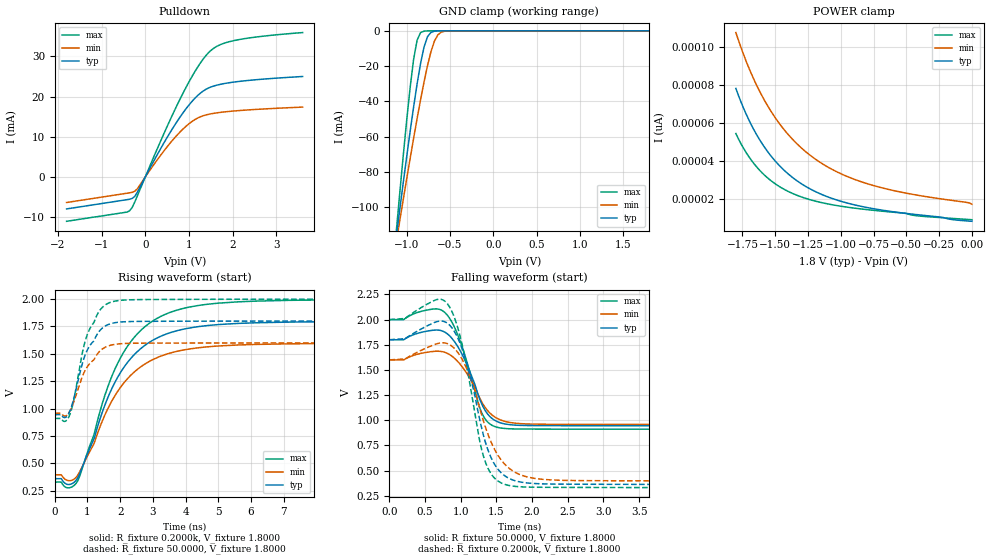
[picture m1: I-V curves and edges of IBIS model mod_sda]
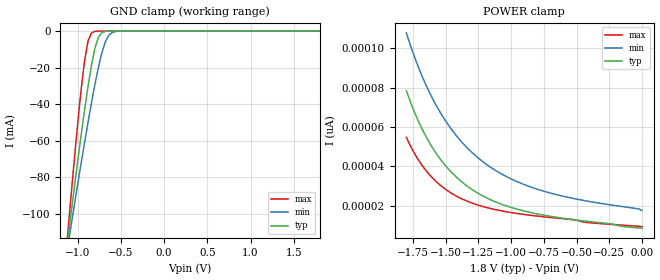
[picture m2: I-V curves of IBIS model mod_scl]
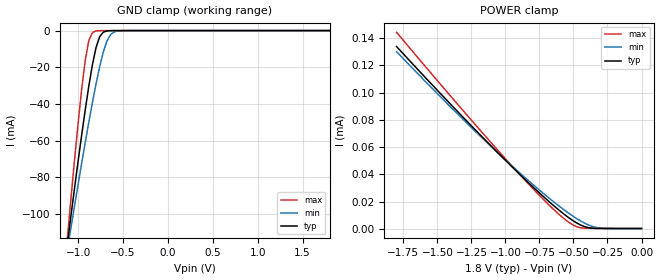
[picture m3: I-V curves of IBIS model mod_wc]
| IBIS (I/O, Buffer, Information, Specification) Model, officially
| electronic behavioral standard for Buffer structures of digital pins.
[IBIS ver]  4.0
[File name] m24m02e_1d8_dfn8.ibs
[File Rev]  1.0
[Date]   10 May 2023
[Source]   CAD & Design Services (Catania) - STMicroelectronics
[Notes]
   (Note1)  This IBIS model includes the DFN8 package parasitic data
   (Note2)  This IBIS model has some Notes about the non-monotonicity
   of the I-V curves, but they are not indicative of problems
   inside the model;
[Disclaimer]
   Customers are solely responsible for all aspects of their
   own product designs or applications using this IBIS Model.
   STMicroelectronics assumes no liability for Custmer Designs
   and applications associated to this IBIS Model.
   In the use of this IBIS Model Customer shall not modify,
   disassemble, alter this Model in whole or in part.
   If Customers do not accept these terms, the IBIS Model
   may not be used. For any problems or modifications please
   contact STMicroelectronics (www.st.com).
[Copyright] (c) 2023 STMicroelectronics
|   Component M24m02e
[Component] M24m02e
[Manufacturer] STMicroelectronics
[Package]
| variable  typ   min   max
R_pkg   0.0   0.0   0.0
L_pkg   0.0H   0.0H   0.0H
C_pkg   0.0F   0.0F   0.0F
[Pin]  signal_name   model_name   R_pin   L_pin   C_pin
1   DU   NC   0.0   0.0   0.0
2   E2   mod_en   0.0   0.0   0.0
3   E3   mod_en   0.0   0.0   0.0
4   VSS   GND   0.0   0.0   0.0
5   SDA   mod_sda   0.0   0.0   0.0
6   SCL   mod_scl   0.0   0.0   0.0
7   WC   mod_wc   0.0   0.0   0.0
8   VCC   POWER   0.0   0.0   0.0
[Package Model]  182694_DFN8   | also called 182694_MLP_2x3
[Define Package Model]  182694_DFN8
[Manufacturer]  STMicroelectronics
[OEM]  STMicroelectronics
[Description]  8 pin DFN8 2x3
[Number Of Pins]  8
[Pin Numbers]
|Pin Num   Terminal Name
1   | net1
2   | net2
3   | net3
4   | net4_GND
5   | net5
6   | net6
7   | net7
8   | net8_VDD
[Model Data]
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[End Model Data]
[End Package Model]
| Models and submodels in the file (4): mod_sda (I/O_open_drain), mod_scl (Input), mod_wc (Input), mod_en (Input)
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|   Model mod_sda
[Model]   mod_sda
Model_type I/O_open_drain
Polarity   Inverting
Enable   Active-High
Vinl   =   0.450V
Vinh   =   1.350V
Vmeas  =   0.900V
Cref   =   30pF
Rref   =   500
Vref   =   1.800V
C_comp   4.636pF   4.427pF   4.855pF
[Temperature Range]   25.0000   85.0000   -40.0000
[Voltage Range]   1.8000V   1.6000V   2.0000V
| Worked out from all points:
|   slope of the pulldown table from 0 to 0.27 V, typ, clamps not added: 49.4 ohm
|   GND clamp passes 1 mA (typ) near -0.72 V on its own axis
|   rising waveform, R_fixture 0.2000k, V_fixture 1.8000: 20-80 % time 1.4ns typ, 1.4ns min, 1.39ns max; typ from 0.36 V to 1.8 V
|   rising waveform, R_fixture 50.0000, V_fixture 1.8000: 20-80 % time 611ps typ, 633ps min, 571ps max; typ from 0.944 V to 1.8 V
|   falling waveform, R_fixture 50.0000, V_fixture 1.8000: 20-80 % time 290ps typ, 309ps min, 271ps max; typ from 1.8 V to 0.944 V
|   falling waveform, R_fixture 0.2000k, V_fixture 1.8000: 20-80 % time 308ps typ, 367ps min, 265ps max; typ from 1.8 V to 0.36 V
[Pulldown]
|Voltage   I(typ)   I(min)   I(max)
-1.8V     -7.942mA   -6.343mA   -11.02mA
-360mV    -5.542mA   -3.943mA   -8.42mA
-240mV    -4.822mA   -3.53mA    -6.215mA
-180mV    -3.76mA    -2.937mA   -4.665mA
420mV     8.349mA    6.387mA    10.62mA
900mV     16.49mA    12.29mA    21.61mA
1.2V      20.27mA    14.66mA    27.34mA
1.38V     21.75mA    15.4mA     30.09mA
1.5V      22.36mA    15.7mA     31.45mA
1.74V     23.09mA    16.09mA    33mA
2.1V      23.7mA     16.47mA    34.06mA
3.6V      24.98mA    17.37mA    35.9mA
[GND_clamp]
|Voltage   I(typ)   I(min)   I(max)
-1.8V     -389.2mA   -332.1mA   -507.3mA
-1.12V    -116.3mA   -119.5mA   -113.3mA
-1.08V    -101mA     -107.4mA   -91.66mA
-1V       -71.13mA   -83.74mA   -50.44mA
-920mV    -42.94mA   -60.76mA   -15.96mA
-880mV    -29.99mA   -49.68mA   -5.261mA
-840mV    -18.43mA   -39.01mA   -1.028mA
-800mV    -9.166mA   -28.93mA   -159.1uA
-760mV    -3.325mA   -19.7mA    -26.96uA
-680mV    -202.6uA   -5.819mA   -1.339uA
-600mV    -10.23uA   -725.2uA   -32.48nA
1.8V      8.512pA    19.96pA    8.401pA
[POWER_clamp]
|Voltage   I(typ)   I(min)   I(max)
-1.8V     78.43pA    107.8pA    54.66pA
-1.74V    67.81pA    96.01pA    46.75pA
-1.68V    58.96pA    85.83pA    40.47pA
-1.62V    51.57pA    77.07pA    35.46pA
-1.54V    43.56pA    67.25pA    30.3pA
-1.46V    37.24pA    59.19pA    26.45pA
-1.38V    32.23pA    52.55pA    23.54pA
-1.2V     24.35pA    41.52pA    19.23pA
-1V       19.06pA    33.56pA    16.45pA
-760mV    15.25pA    27.51pA    14.36pA
-500mV    12.65pA    23.3pA     12.6pA
0V        8.512pA    17.5pA     9.335pA
[Ramp]
| variable   typ   min   max
dV/dt_r  0.5134/0.6085n   0.3853/0.6461n   0.6541/0.5659n
dV/dt_f  0.5133/0.3737n   0.3852/0.3840n   0.6540/0.3349n
R_load = 50.0000
[Rising Waveform]
R_fixture= 0.2000k
V_fixture= 1.8000
V_fixture_min= 1.6000
V_fixture_max= 2.0000
|time   V(typ)   V(min)   V(max)
0s        359.6mV    394.7mV    328.2mV
420ps     306mV      340.8mV    275.4mV
690ps     360.9mV    386.1mV    333.9mV
1.19ns    714mV      672.4mV    753.6mV
1.57ns    1.061V     966.2mV    1.155V
1.91ns    1.279V     1.151V     1.406V
2.45ns    1.499V     1.339V     1.658V
3.13ns    1.645V     1.465V     1.824V
5.04ns    1.768V     1.572V     1.964V
10ns      1.796V     1.596V     1.996V
[Rising Waveform]
R_fixture= 50.0000
V_fixture= 1.8000
V_fixture_min= 1.6000
V_fixture_max= 2.0000
|time   V(typ)   V(min)   V(max)
0s        943.9mV    957.6mV    909.6mV
300ps     917.2mV    931.5mV    882.2mV
430ps     955.9mV    959.9mV    923.2mV
550ps     1.056V     1.036V     1.036V
830ps     1.398V     1.282V     1.49V
990ps     1.532V     1.38V      1.672V
1.37ns    1.71V      1.522V     1.894V
1.69ns    1.774V     1.577V     1.969V
2.61ns    1.796V     1.597V     1.995V
10ns      1.8V       1.6V       2V
[Falling Waveform]
R_fixture= 50.0000
V_fixture= 1.8000
V_fixture_min= 1.6000
V_fixture_max= 2.0000
|time   V(typ)   V(min)   V(max)
0s        1.8V       1.6V       2V
200ps     1.8V       1.6V       2V
600ps     1.894V     1.683V     2.104V
780ps     1.874V     1.675V     2.068V
980ps     1.706V     1.566V     1.809V
1.3ns     1.153V     1.174V     1.065V
1.4ns     1.043V     1.077V     968mV
1.56ns    973.7mV    1.003V     923.2mV
2.18ns    946.3mV    960.3mV    912.1mV
10ns      944.1mV    957.8mV    909.8mV
[Falling Waveform]
R_fixture= 0.2000k
V_fixture= 1.8000
V_fixture_min= 1.6000
V_fixture_max= 2.0000
|time   V(typ)   V(min)   V(max)
0s        1.8V       1.6V       2V
660ps     1.979V     1.759V     2.199V
820ps     1.96V      1.76V      2.151V
940ps     1.844V     1.691V     1.961V
1.06ns    1.623V     1.55V      1.618V
1.34ns    794.8mV    944.2mV    595.4mV
1.48ns    555.5mV    702.5mV    420.8mV
1.66ns    428.9mV    533.6mV    354.7mV
2.46ns    365.1mV    402.8mV    333mV
10ns      360.1mV    395.3mV    328.6mV
|   Model mod_scl
[Model]   mod_scl
Model_type Input
Vinl   =   0.6500V
Vinh   =   1.2000V
C_comp   3.062pF   2.925pF   3.207pF
[Temperature Range]  25.0000   85.0000   -40.0000
[Voltage Range]   1.8000V   1.6000V   2.0000V
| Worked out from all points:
|   GND clamp passes 1 mA (typ) near -0.72 V on its own axis
[GND_clamp]
|Voltage   I(typ)   I(min)   I(max)
-1.8V     -389.2mA   -332.1mA   -507.3mA
-1.12V    -116.3mA   -119.5mA   -113.3mA
-1.08V    -101mA     -107.4mA   -91.66mA
-1V       -71.13mA   -83.74mA   -50.44mA
-920mV    -42.94mA   -60.76mA   -15.96mA
-880mV    -29.99mA   -49.68mA   -5.261mA
-840mV    -18.43mA   -39.01mA   -1.028mA
-800mV    -9.166mA   -28.93mA   -159.1uA
-760mV    -3.325mA   -19.7mA    -26.96uA
-680mV    -202.6uA   -5.819mA   -1.339uA
-600mV    -10.23uA   -725.2uA   -32.48nA
1.8V      8.512pA    19.96pA    8.401pA
[POWER_clamp]
|Voltage   I(typ)   I(min)   I(max)
-1.8V     78.43pA    107.8pA    54.66pA
-1.74V    67.81pA    96.01pA    46.75pA
-1.68V    58.96pA    85.83pA    40.47pA
-1.62V    51.57pA    77.07pA    35.46pA
-1.54V    43.56pA    67.25pA    30.3pA
-1.46V    37.24pA    59.19pA    26.45pA
-1.38V    32.23pA    52.55pA    23.54pA
-1.2V     24.35pA    41.52pA    19.23pA
-1V       19.06pA    33.56pA    16.45pA
-760mV    15.25pA    27.51pA    14.36pA
-500mV    12.65pA    23.3pA     12.6pA
0V        8.512pA    17.5pA     9.335pA
|   Model mod_wc
[Model]   mod_wc
Model_type Input
Vinl   =   0.6500V
Vinh   =   1.2000V
C_comp   3.062pF   2.925pF   3.207pF
[Temperature Range]  25.0000   85.0000   -40.0000
[Voltage Range]   1.8000V   1.6000V   2.0000V
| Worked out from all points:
|   GND clamp passes 1 mA (typ) near -0.72 V on its own axis
[GND_clamp]
|Voltage   I(typ)   I(min)   I(max)
-1.8V     -389.2mA   -332.1mA   -507.3mA
-1.12V    -116.3mA   -119.5mA   -113.3mA
-1.08V    -101mA     -107.5mA   -91.66mA
-1V       -71.13mA   -83.75mA   -50.44mA
-920mV    -42.94mA   -60.76mA   -15.97mA
-880mV    -30mA      -49.68mA   -5.271mA
-840mV    -18.44mA   -39.01mA   -1.042mA
-800mV    -9.172mA   -28.93mA   -174.8uA
-760mV    -3.333mA   -19.7mA    -43.28uA
-680mV    -214.5uA   -5.824mA   -16.74uA
-600mV    -21.97uA   -733.4uA   -11.84uA
1.8V      2.23uA     1.139uA    2.602uA
[POWER_clamp]
|Voltage   I(typ)   I(min)   I(max)
-1.8V     133.9uA    130.1uA    144.3uA
-1.4V     91.22uA    89.2uA     97.16uA
-1.08V    58.33uA    58.11uA    60.44uA
-760mV    27.26uA    29.3uA     25.61uA
-640mV    16.58uA    19.41uA    13.72uA
-560mV    10.08uA    13.28uA    6.727uA
-500mV    5.808uA    9.072uA    2.651uA
-460mV    3.444uA    6.532uA    1.072uA
-400mV    1.101uA    3.328uA    446.9nA
-340mV    348.6nA    1.216uA    402.7nA
-260mV    234.9nA    259.7nA    400.3nA
0V        229.3nA    138.9nA    400.3nA
